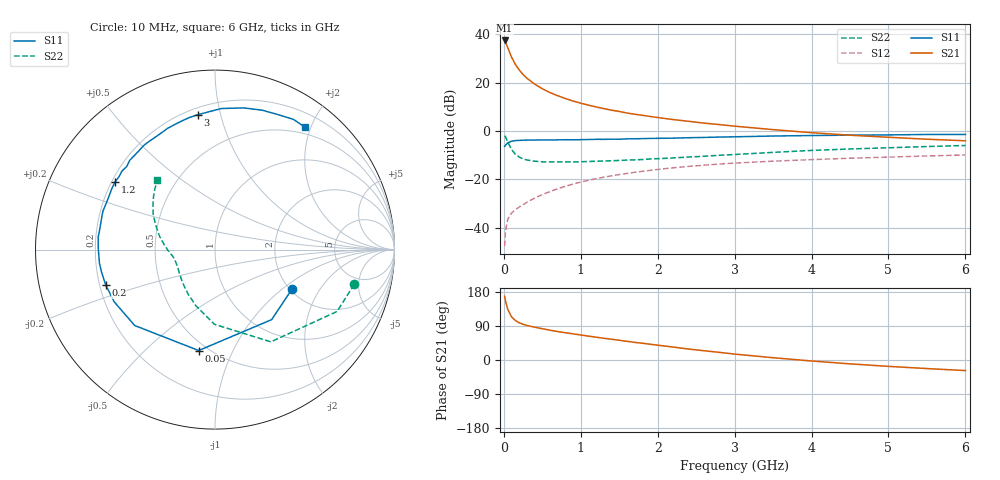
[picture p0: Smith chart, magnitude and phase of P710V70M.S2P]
! SIEMENS Small Signal Semiconductors
! BFP196
! Si NPN RF Bipolar Junction Transistor in SOT143
! VCE = 10 V  IC = 70 mA
! Common Emitter S-Parameters:  May  1996
# GHz  S  MA  R  50
!  f  S11  S21  S12  S22
! GHz  MAG  ANG  MAG  ANG  MAG  ANG  MAG  ANG
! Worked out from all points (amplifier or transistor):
!   36 points, 10 MHz to 6 GHz, reference 50 ohm
!   highest |S21| = 37.4 dB at 10 MHz (marker M1)
!   |S21| within 3 dB of that: start of sweep to 51.37 MHz
!   unconditionally stable (mu >= 1): 478.9 MHz to 4.996 GHz
!   at 250 MHz: K = 0.82, MSG = 26.8 dB, |S12| = -30.4 dB
!   at 1.4 GHz: K = 1.09, MAG = 11.7 dB, |S12| = -18.5 dB
!   at 6 GHz: K = 0.98, MSG = 2.9 dB, |S12| = -9.9 dB
!   S11 on the Smith chart (normalised r, x): 10 MHz: 2.07, -1.17; 50 MHz: 0.45, -0.75; 200 MHz: 0.22, -0.15; 1.2 GHz: 0.21, +0.29; 3 GHz: 0.24, +0.85; 6 GHz: 0.40, +1.91
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0.01  0.4824 -26.7  73.73 168.2  0.0042 69.0  0.7998 -14.0
0.02  0.502 -51.0  69 156.9  0.0082 66.2  0.7622 -26.9
0.05  0.5696 -99.2  52.86 133.8  0.015 53.7  0.6009 -58.8
0.1  0.6156 -136.6  33.44 114.0  0.0202 46.7  0.4161 -90.4
0.15  0.6325 -152.6  23.63 104.2  0.024 46.9  0.3301 -108.9
0.2  0.6401 -162.0  18.17 98.3  0.0269 49.7  0.2896 -121.2
0.25  0.6443 -168.7  14.6 94.2  0.0302 51.8  0.2651 -130.7
0.3  0.6485 -173.2  12.27 91.2  0.0338 54.4  0.2525 -137.0
0.4  0.6502 179.5  9.282 86.6  0.0413 58.1  0.2378 -146.6
0.5  0.6544 174.0  7.43 82.5  0.0485 60.1  0.2311 -152.9
0.6  0.652 169.2  6.197 78.7  0.0563 60.7  0.2293 -157.0
0.7  0.6556 164.6  5.335 75.0  0.0642 61.2  0.2293 -160.4
0.9  0.6587 157.0  4.148 69.0  0.0803 60.2  0.2299 -165.2
1.1  0.6674 149.6  3.412 63.0  0.0959 58.7  0.235 -168.6
1.2  0.6723 146.1  3.132 60.2  0.1037 57.9  0.2373 -170.2
1.6  0.6881 133.6  2.349 49.3  0.133 52.7  0.2506 -175.6
2.2  0.7113 116.7  1.721 34.2  0.1737 44.0  0.2775 176.4
3  0.7579 97.2  1.257 15.6  0.2178 32.4  0.3271 164.1
3.5  0.7869 87.4  1.067 6.0  0.2383 25.5  0.3618 156.7
4.5  0.8202 71.2  0.817 -10.2  0.274 13.9  0.425 144.4
5.5  0.8468 59.0  0.676 -22.6  0.305 3.4  0.4774 134.5
6  0.8467 53.6  0.628 -27.9  0.3197 -2.2  0.5018 129.7
